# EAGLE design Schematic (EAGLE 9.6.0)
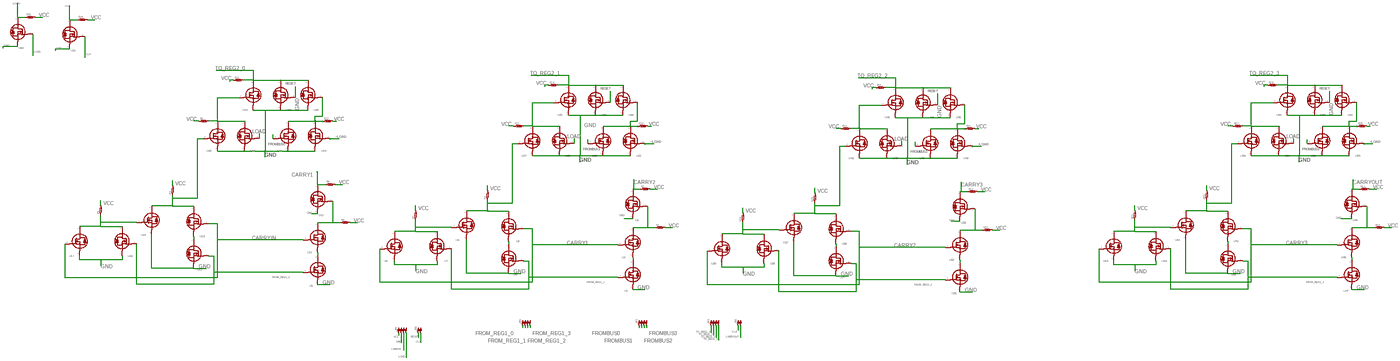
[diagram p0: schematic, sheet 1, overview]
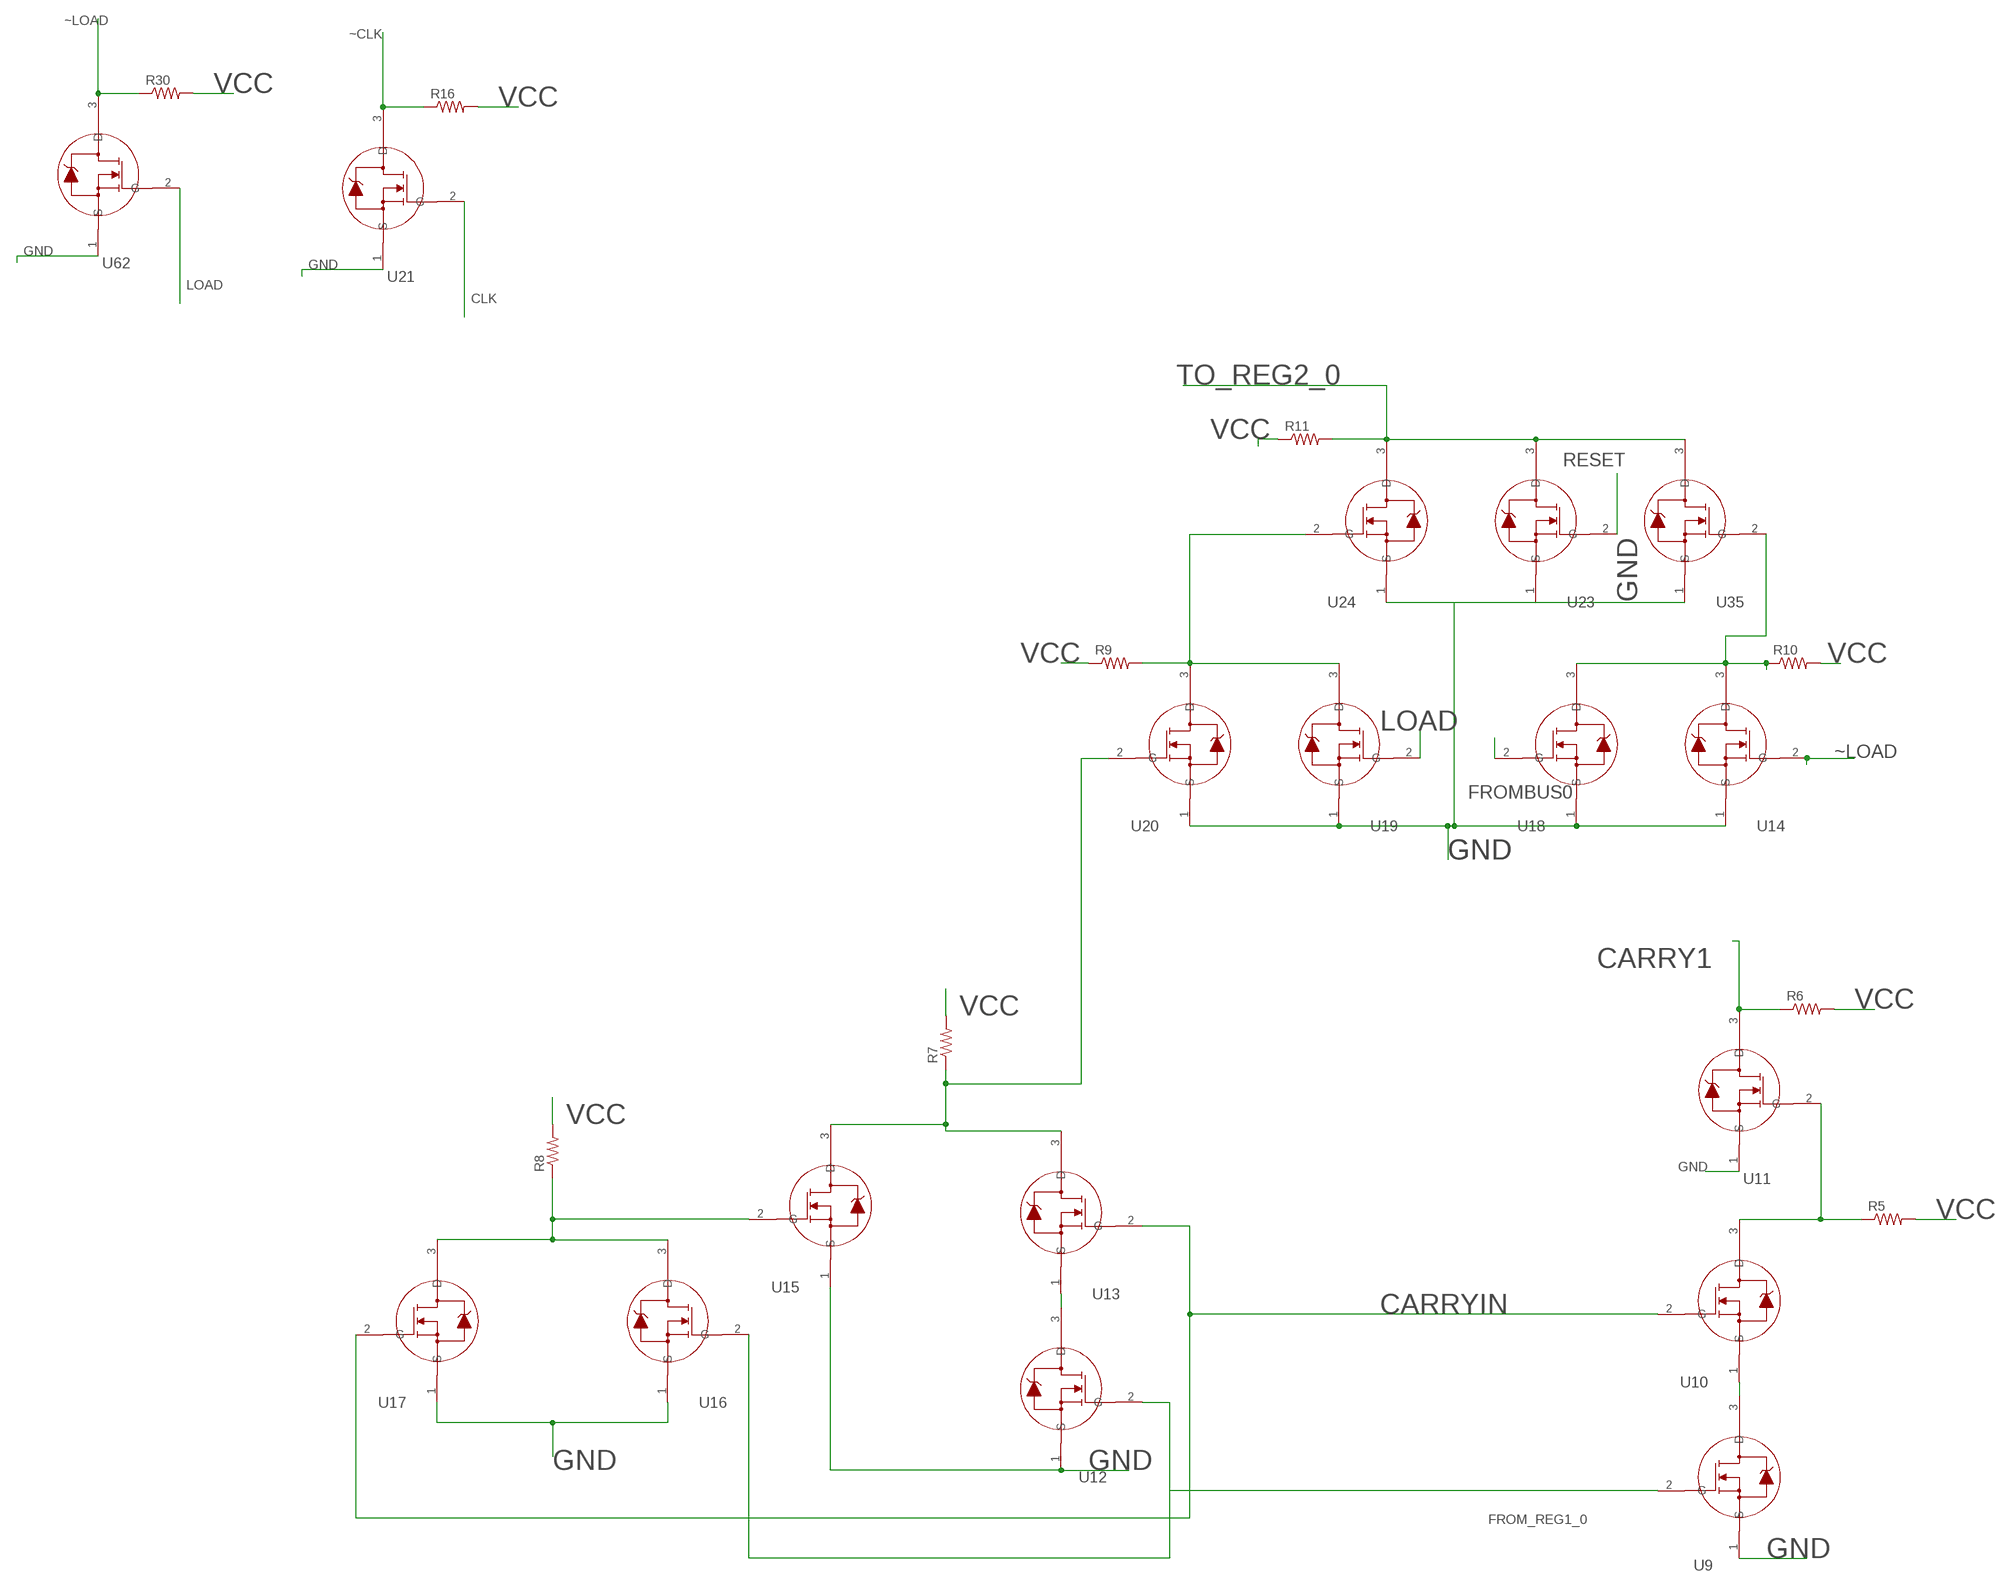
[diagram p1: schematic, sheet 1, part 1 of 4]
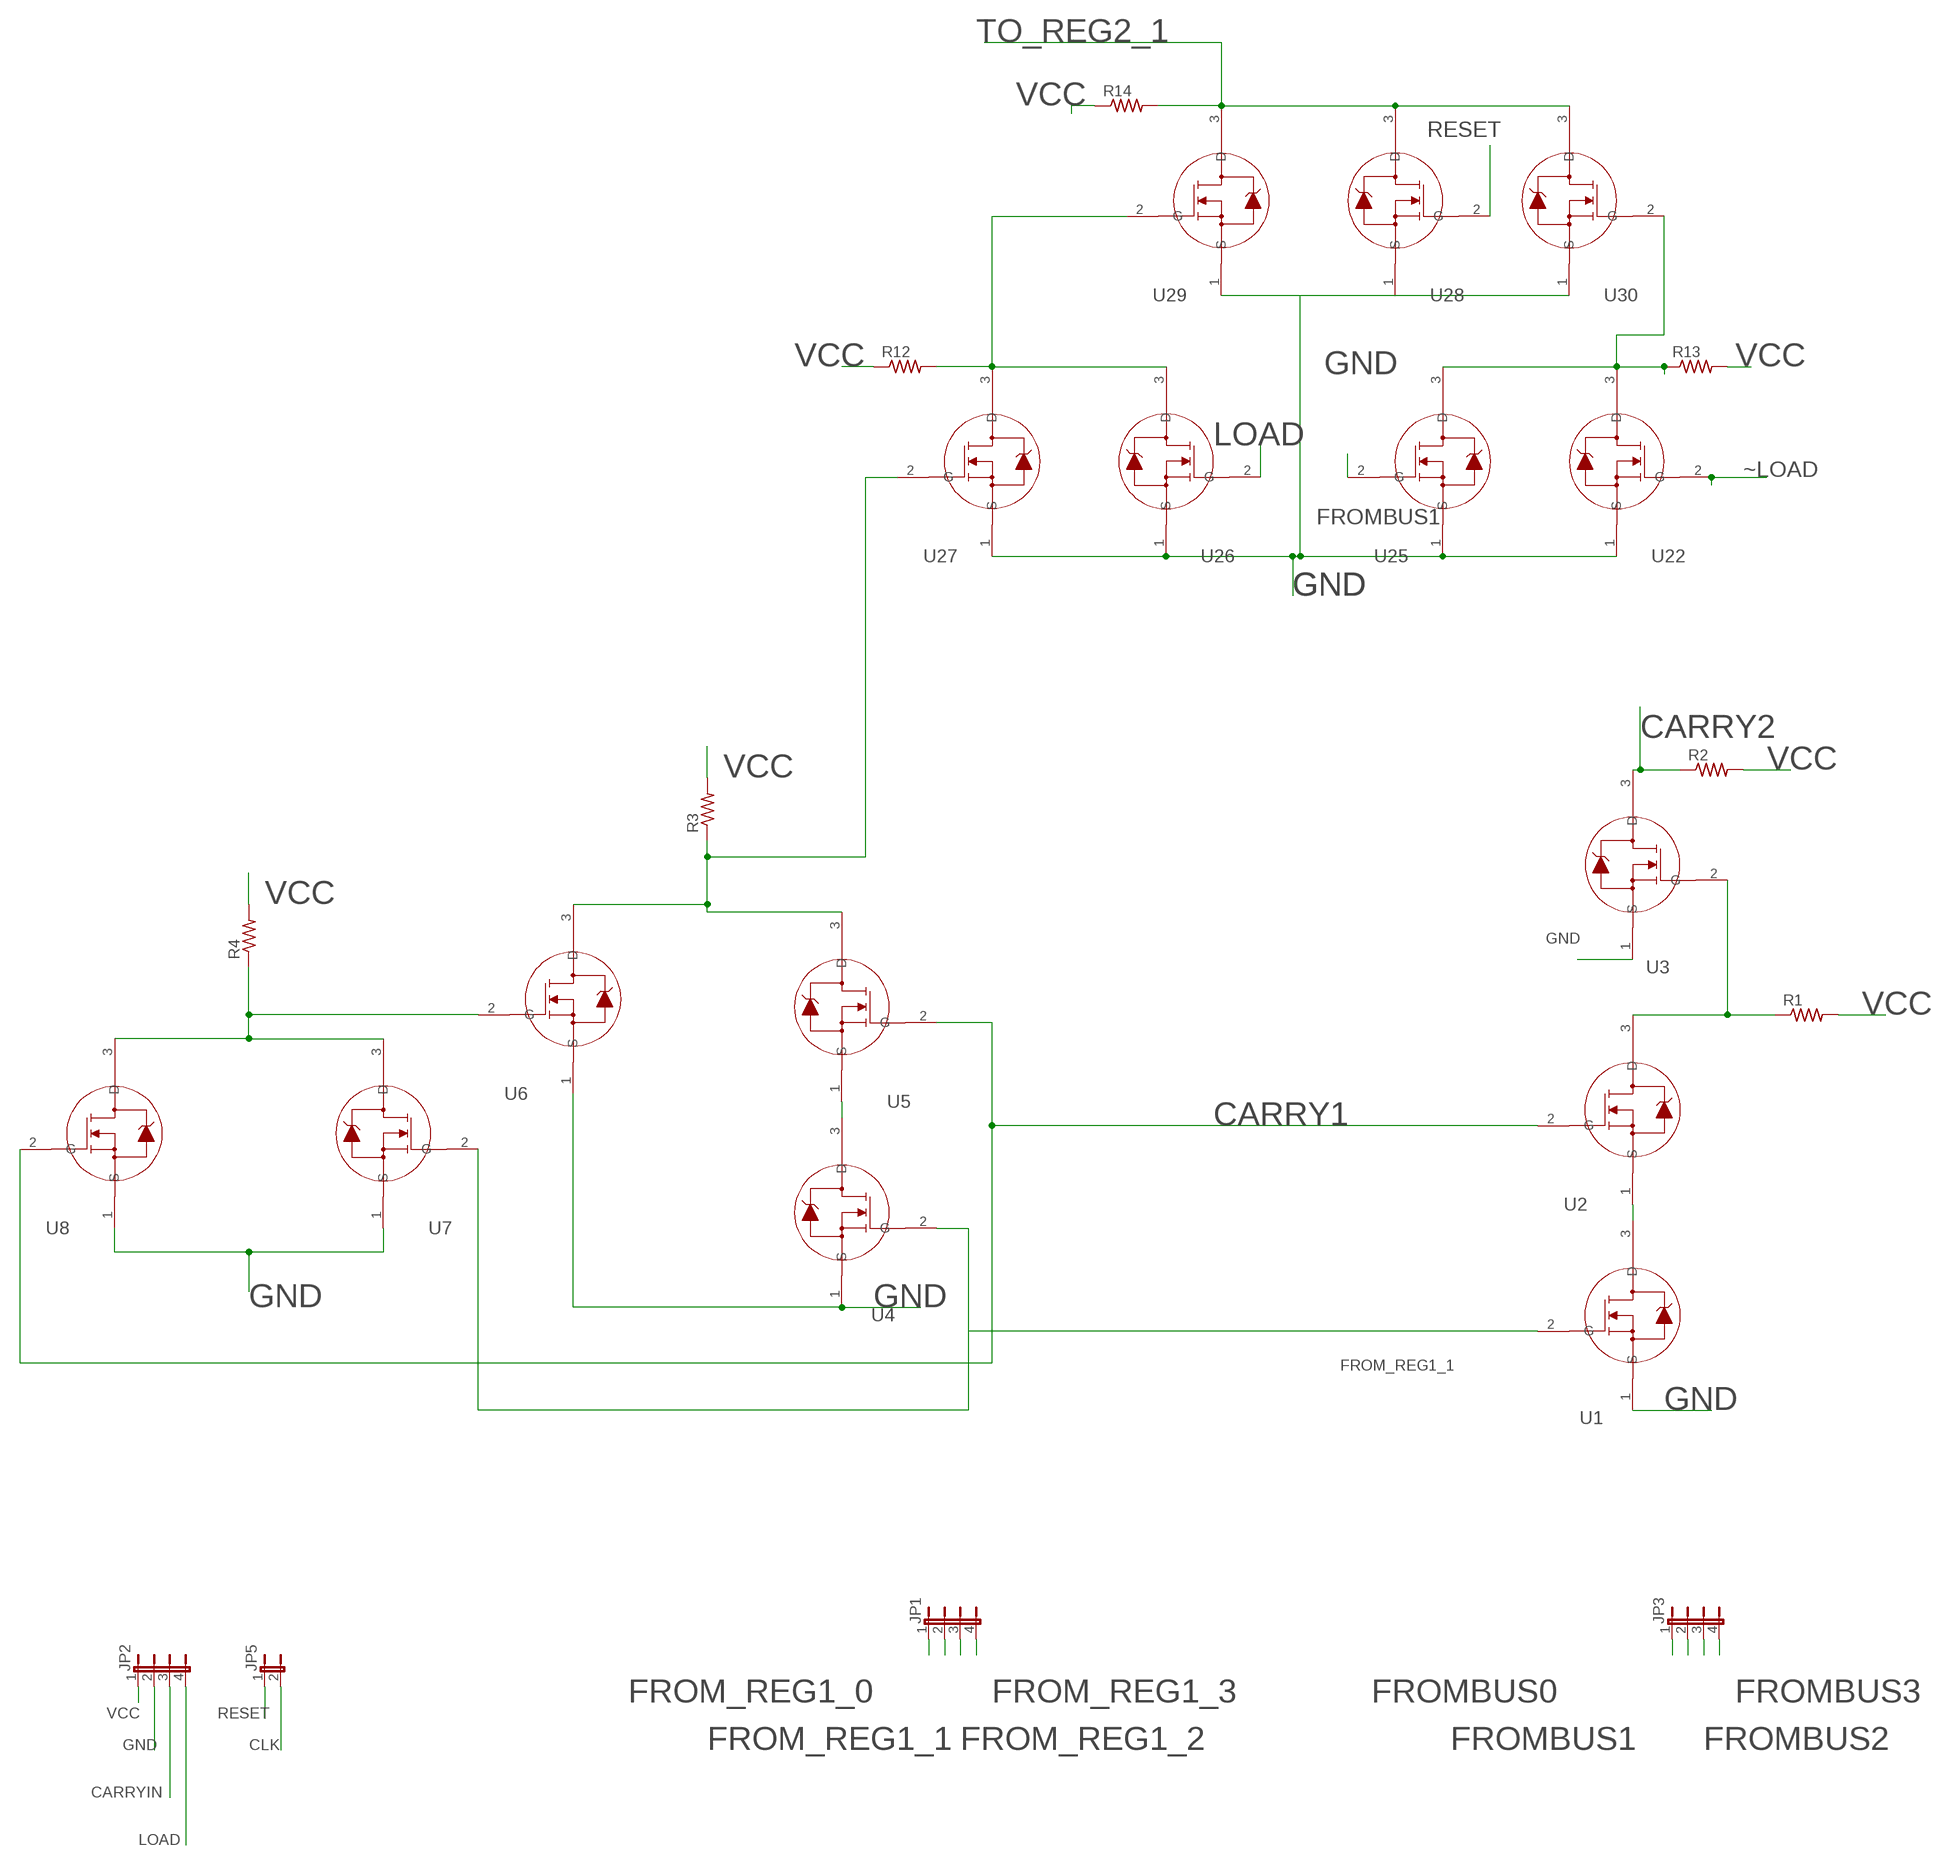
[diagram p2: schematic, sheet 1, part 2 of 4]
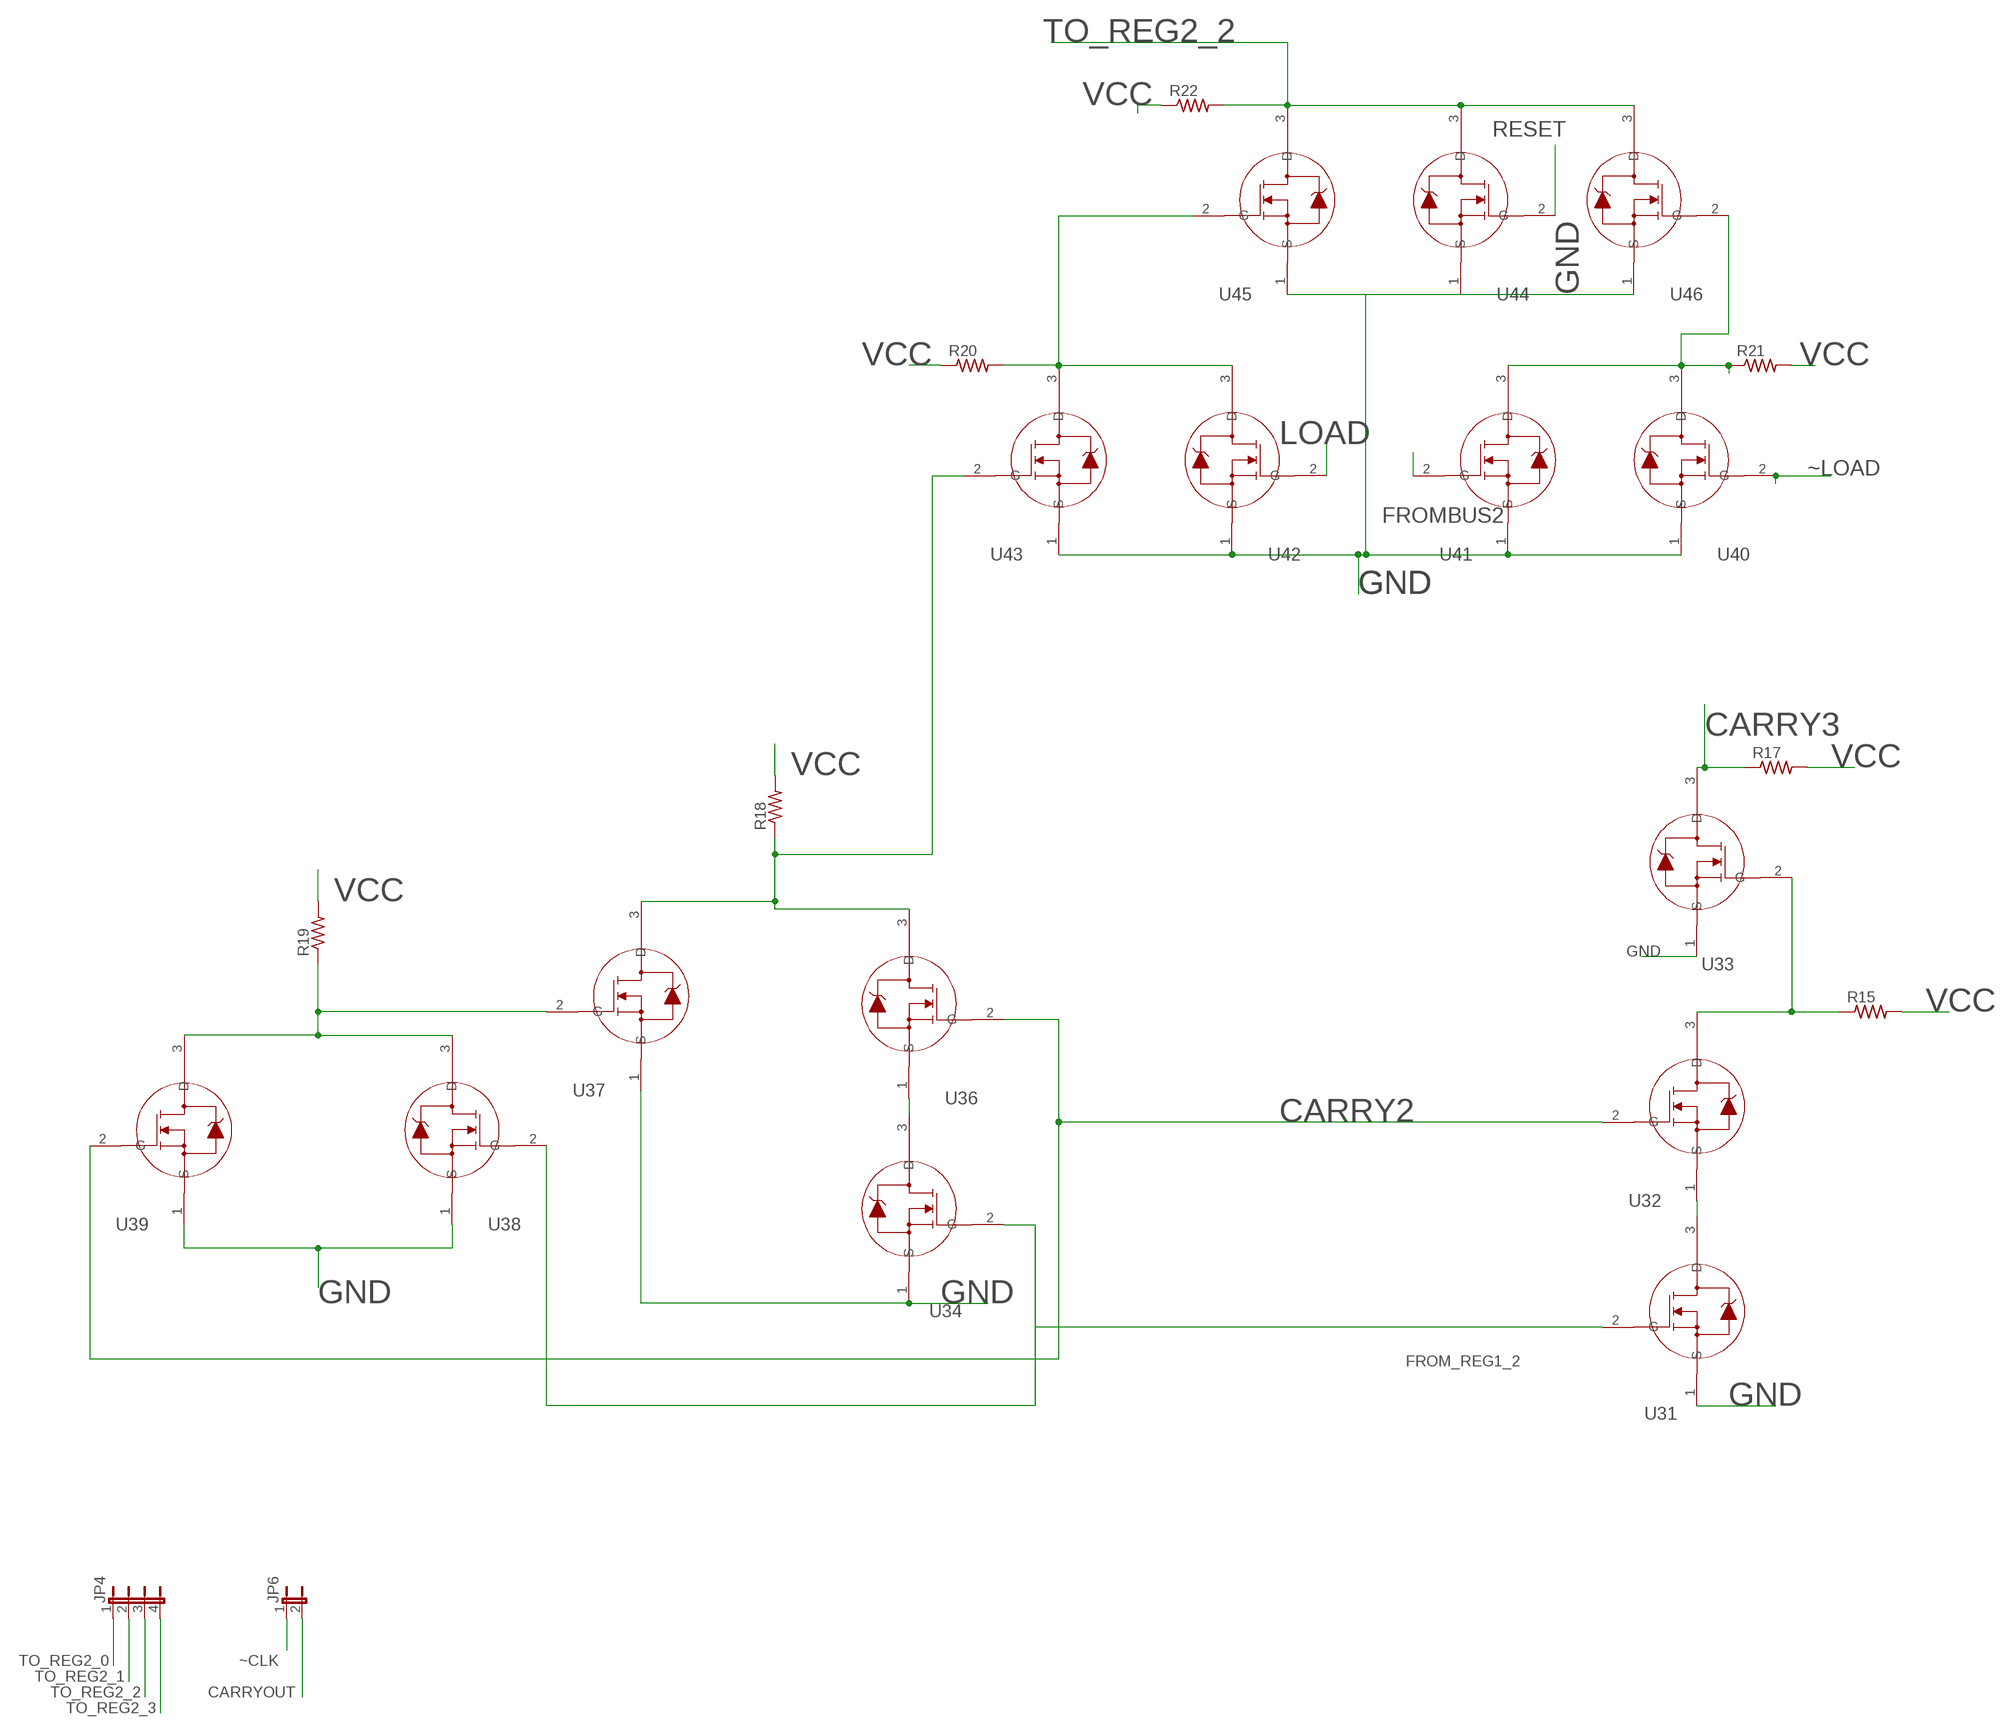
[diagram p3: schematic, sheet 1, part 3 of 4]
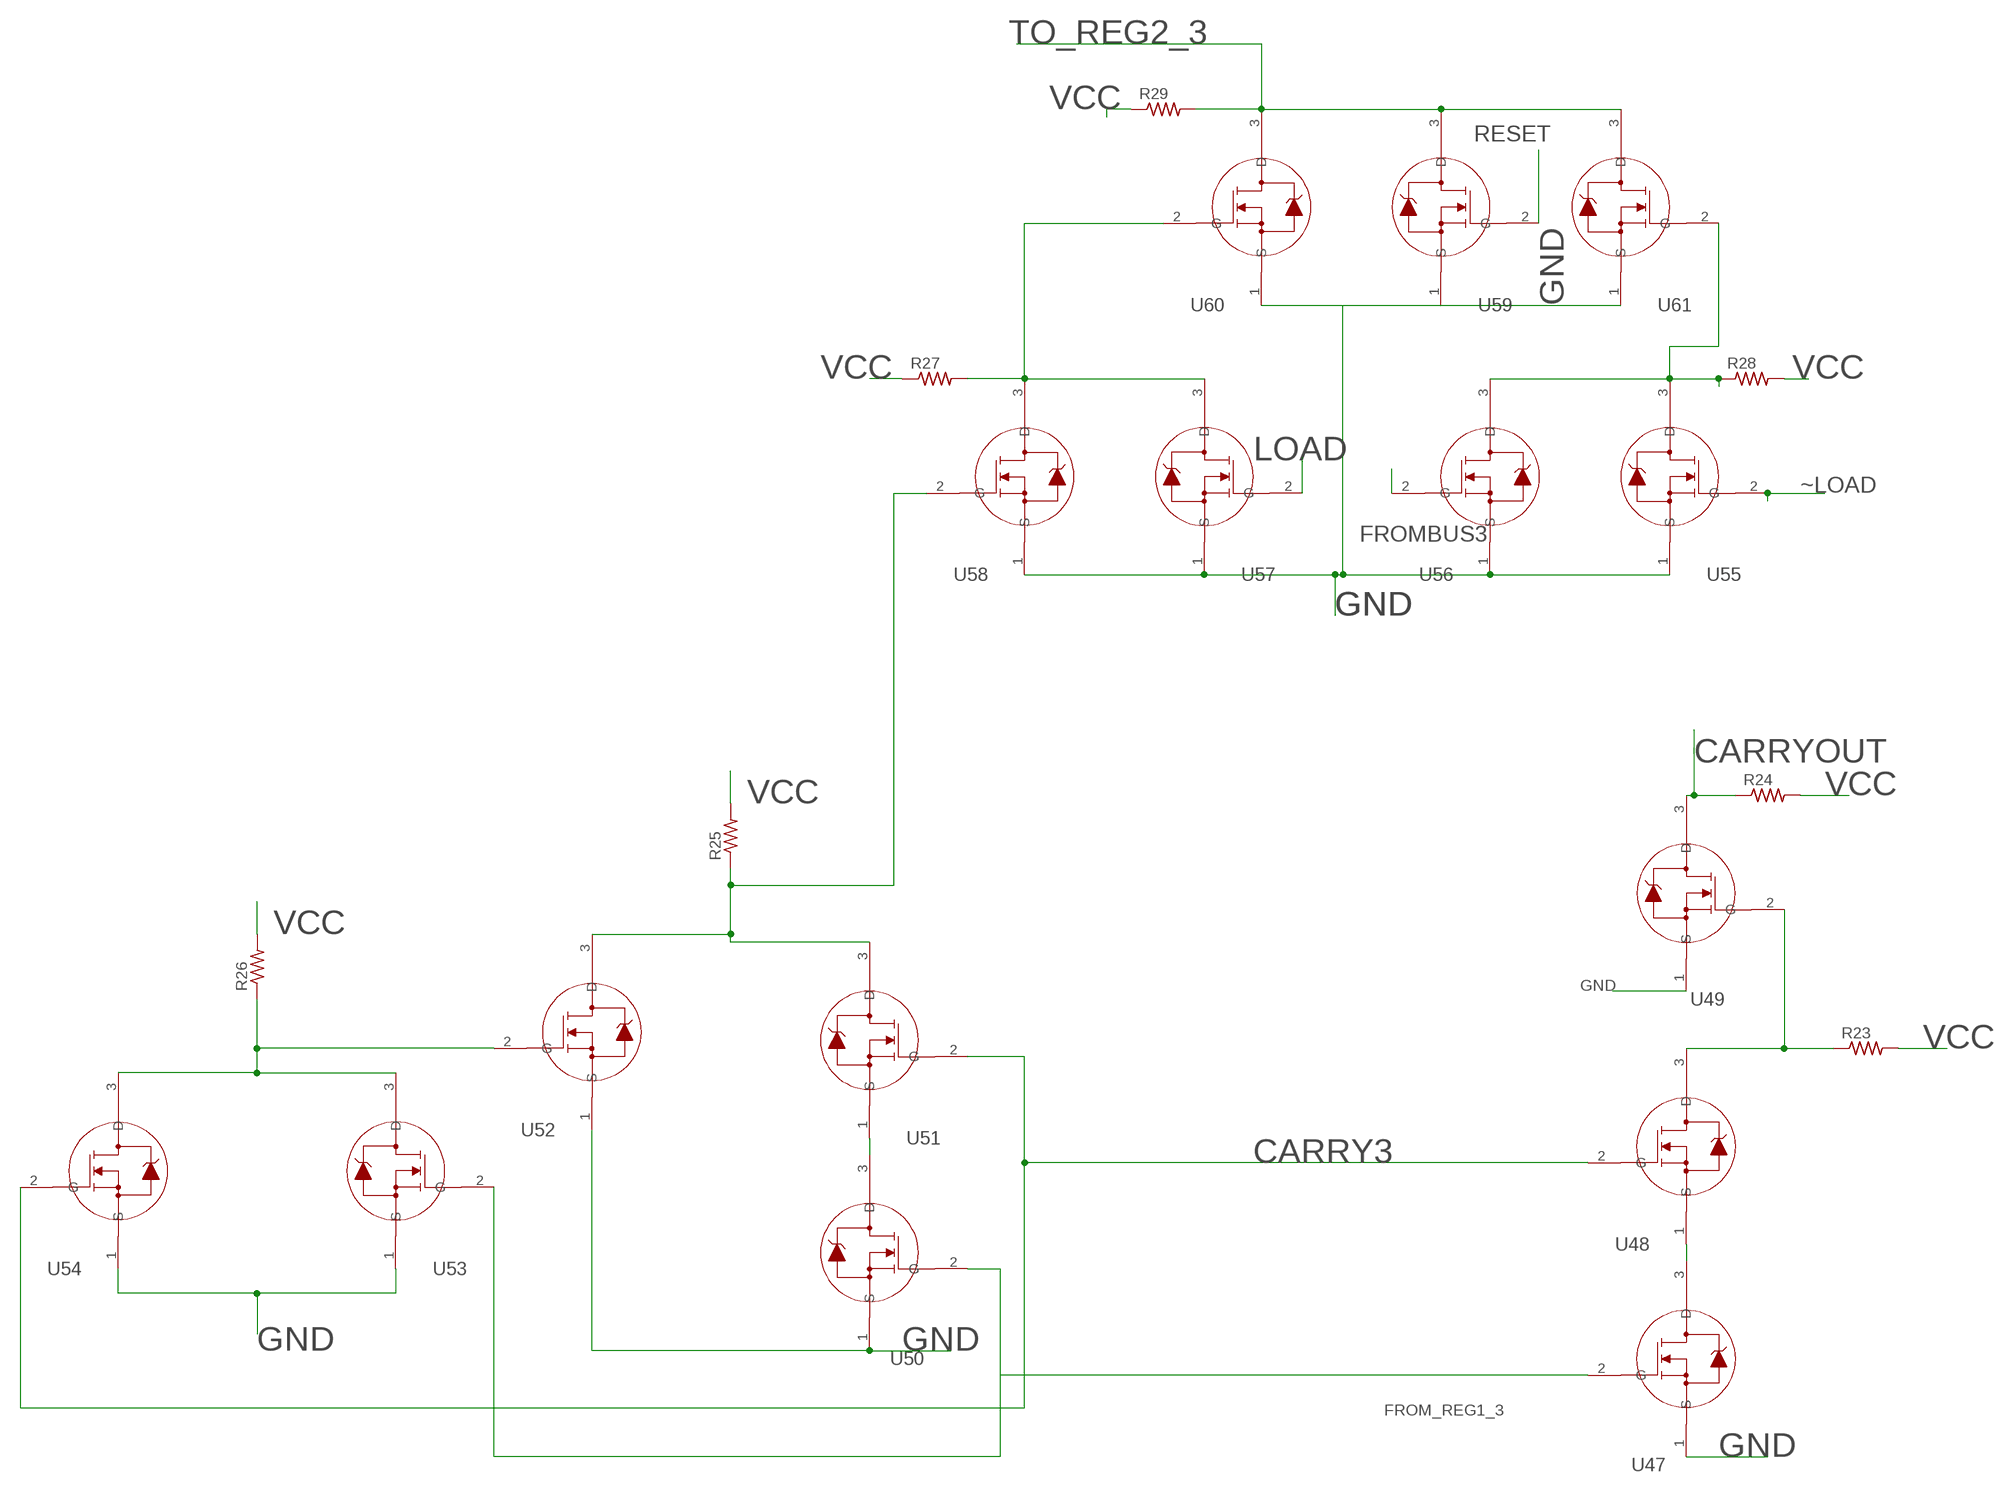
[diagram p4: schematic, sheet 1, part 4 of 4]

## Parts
JP1  JP4E  [JP4]
JP2  JP4E  [JP4]
JP3  JP4E  [JP4]
JP4  JP4E  [JP4]
JP5  JP1E  [JP1]
JP6  JP1E  [JP1]
R1  R-US_0204/7  [0204/7]
R2  R-US_0204/7  [0204/7]
R3  R-US_0204/7  [0204/7]
R4  R-US_0204/7  [0204/7]
R5  R-US_0204/7  [0204/7]
R6  R-US_0204/7  [0204/7]
R7  R-US_0204/7  [0204/7]
R8  R-US_0204/7  [0204/7]
R9  R-US_0204/7  [0204/7]
R10  R-US_0204/7  [0204/7]
R11  R-US_0204/7  [0204/7]
R12  R-US_0204/7  [0204/7]
R13  R-US_0204/7  [0204/7]
R14  R-US_0204/7  [0204/7]
R15  R-US_0204/7  [0204/7]
R16  R-US_0204/7  [0204/7]
R17  R-US_0204/7  [0204/7]
R18  R-US_0204/7  [0204/7]
R19  R-US_0204/7  [0204/7]
R20  R-US_0204/7  [0204/7]
R21  R-US_0204/7  [0204/7]
R22  R-US_0204/7  [0204/7]
R23  R-US_0204/7  [0204/7]
R24  R-US_0204/7  [0204/7]
R25  R-US_0204/7  [0204/7]
R26  R-US_0204/7  [0204/7]
R27  R-US_0204/7  [0204/7]
R28  R-US_0204/7  [0204/7]
R29  R-US_0204/7  [0204/7]
R30  R-US_0204/7  [0204/7]
U1  2N7000RLRAG  [TO-92_ONS]
U2  2N7000RLRAG  [TO-92_ONS]
U3  2N7000RLRAG  [TO-92_ONS]
U4  2N7000RLRAG  [TO-92_ONS]
U5  2N7000RLRAG  [TO-92_ONS]
U6  2N7000RLRAG  [TO-92_ONS]
U7  2N7000RLRAG  [TO-92_ONS]
U8  2N7000RLRAG  [TO-92_ONS]
U9  2N7000RLRAG  [TO-92_ONS]
U10  2N7000RLRAG  [TO-92_ONS]
U11  2N7000RLRAG  [TO-92_ONS]
U12  2N7000RLRAG  [TO-92_ONS]
U13  2N7000RLRAG  [TO-92_ONS]
U14  2N7000RLRAG  [TO-92_ONS]
U15  2N7000RLRAG  [TO-92_ONS]
U16  2N7000RLRAG  [TO-92_ONS]
U17  2N7000RLRAG  [TO-92_ONS]
U18  2N7000RLRAG  [TO-92_ONS]
U19  2N7000RLRAG  [TO-92_ONS]
U20  2N7000RLRAG  [TO-92_ONS]
U21  2N7000RLRAG  [TO-92_ONS]
U22  2N7000RLRAG  [TO-92_ONS]
U23  2N7000RLRAG  [TO-92_ONS]
U24  2N7000RLRAG  [TO-92_ONS]
U25  2N7000RLRAG  [TO-92_ONS]
U26  2N7000RLRAG  [TO-92_ONS]
U27  2N7000RLRAG  [TO-92_ONS]
U28  2N7000RLRAG  [TO-92_ONS]
U29  2N7000RLRAG  [TO-92_ONS]
U30  2N7000RLRAG  [TO-92_ONS]
U31  2N7000RLRAG  [TO-92_ONS]
U32  2N7000RLRAG  [TO-92_ONS]
U33  2N7000RLRAG  [TO-92_ONS]
U34  2N7000RLRAG  [TO-92_ONS]
U35  2N7000RLRAG  [TO-92_ONS]
U36  2N7000RLRAG  [TO-92_ONS]
U37  2N7000RLRAG  [TO-92_ONS]
U38  2N7000RLRAG  [TO-92_ONS]
U39  2N7000RLRAG  [TO-92_ONS]
U40  2N7000RLRAG  [TO-92_ONS]
U41  2N7000RLRAG  [TO-92_ONS]
U42  2N7000RLRAG  [TO-92_ONS]
U43  2N7000RLRAG  [TO-92_ONS]
U44  2N7000RLRAG  [TO-92_ONS]
U45  2N7000RLRAG  [TO-92_ONS]
U46  2N7000RLRAG  [TO-92_ONS]
U47  2N7000RLRAG  [TO-92_ONS]
U48  2N7000RLRAG  [TO-92_ONS]
U49  2N7000RLRAG  [TO-92_ONS]
U50  2N7000RLRAG  [TO-92_ONS]
U51  2N7000RLRAG  [TO-92_ONS]
U52  2N7000RLRAG  [TO-92_ONS]
U53  2N7000RLRAG  [TO-92_ONS]
U54  2N7000RLRAG  [TO-92_ONS]
U55  2N7000RLRAG  [TO-92_ONS]
U56  2N7000RLRAG  [TO-92_ONS]
U57  2N7000RLRAG  [TO-92_ONS]
U58  2N7000RLRAG  [TO-92_ONS]
U59  2N7000RLRAG  [TO-92_ONS]
U60  2N7000RLRAG  [TO-92_ONS]
U61  2N7000RLRAG  [TO-92_ONS]
U62  2N7000RLRAG  [TO-92_ONS]

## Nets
CARRY1: R6.1 U2.2(G) U5.2(G) U8.2(G) U11.3(D)
CARRY2: R2.1 U3.3(D) U32.2(G) U36.2(G) U39.2(G)
CARRY3: R17.1 U33.3(D) U48.2(G) U51.2(G) U54.2(G)
CARRYIN: JP2.3 U10.2(G) U13.2(G) U17.2(G)
CARRYOUT: JP6.2 R24.1 U49.3(D)
CLK: JP5.2 U21.2(G)
FROM_REG1_0: JP1.1 U9.2(G) U12.2(G) U16.2(G)
FROM_REG1_1: JP1.2 U1.2(G) U4.2(G) U7.2(G)
FROM_REG1_2: JP1.3 U31.2(G) U34.2(G) U38.2(G)
FROM_REG1_3: JP1.4 U47.2(G) U50.2(G) U53.2(G)
FROMBUS0: JP3.1 U18.2(G)
FROMBUS1: JP3.2 U25.2(G)
FROMBUS2: JP3.3 U41.2(G)
FROMBUS3: JP3.4 U56.2(G)
GND: JP2.2 U1.1(S) U3.1(S) U4.1(S) U6.1(S) U7.1(S) U8.1(S) U9.1(S) U11.1(S) U12.1(S) U14.1(S) U15.1(S) U16.1(S) U17.1(S) U18.1(S) U19.1(S) U20.1(S) U21.1(S) U22.1(S) U23.1(S) U24.1(S) U25.1(S) U26.1(S) U27.1(S) U28.1(S) U29.1(S) U30.1(S) U31.1(S) U33.1(S) U34.1(S) U35.1(S) U37.1(S) U38.1(S) U39.1(S) U40.1(S) U41.1(S) U42.1(S) U43.1(S) U44.1(S) U45.1(S) U46.1(S) U47.1(S) U49.1(S) U50.1(S) U52.1(S) U53.1(S) U54.1(S) U55.1(S) U56.1(S) U57.1(S) U58.1(S) U59.1(S) U60.1(S) U61.1(S) U62.1(S)
LOAD: JP2.4 U19.2(G) U26.2(G) U42.2(G) U57.2(G) U62.2(G)
N$1: U1.3(D) U2.1(S)
N$2: R1.1 U2.3(D) U3.2(G)
N$3: U31.3(D) U32.1(S)
N$4: U4.3(D) U5.1(S)
N$5: R3.1 U5.3(D) U6.3(D) U27.2(G)
N$6: R4.1 U6.2(G) U7.3(D) U8.3(D)
N$7: R12.2 U26.3(D) U27.3(D) U29.2(G)
N$8: R13.1 U22.3(D) U25.3(D) U30.2(G)
N$9: R9.2 U19.3(D) U20.3(D) U24.2(G)
N$10: U9.3(D) U10.1(S)
N$11: R15.1 U32.3(D) U33.2(G)
N$12: R5.1 U10.3(D) U11.2(G)
N$13: U12.3(D) U13.1(S)
N$15: R7.1 U13.3(D) U15.3(D) U20.2(G)
N$16: R8.1 U15.2(G) U16.3(D) U17.3(D)
N$17: R10.1 U14.3(D) U18.3(D) U35.2(G)
N$18: U47.3(D) U48.1(S)
N$19: R23.1 U48.3(D) U49.2(G)
N$20: U34.3(D) U36.1(S)
N$21: R18.1 U36.3(D) U37.3(D) U43.2(G)
N$22: R19.1 U37.2(G) U38.3(D) U39.3(D)
N$23: R20.2 U42.3(D) U43.3(D) U45.2(G)
N$24: R21.1 U40.3(D) U41.3(D) U46.2(G)
N$25: U50.3(D) U51.1(S)
N$26: R25.1 U51.3(D) U52.3(D) U58.2(G)
N$27: R26.1 U52.2(G) U53.3(D) U54.3(D)
N$28: R27.2 U57.3(D) U58.3(D) U60.2(G)
N$29: R28.1 U55.3(D) U56.3(D) U61.2(G)
RESET: JP5.1 U23.2(G) U28.2(G) U44.2(G) U59.2(G)
TO_REG2_0: JP4.1 R11.2 U23.3(D) U24.3(D) U35.3(D)
TO_REG2_1: JP4.2 R14.2 U28.3(D) U29.3(D) U30.3(D)
TO_REG2_2: JP4.3 R22.2 U44.3(D) U45.3(D) U46.3(D)
TO_REG2_3: JP4.4 R29.2 U59.3(D) U60.3(D) U61.3(D)
VCC: JP2.1 R1.2 R2.2 R3.2 R4.2 R5.2 R6.2 R7.2 R8.2 R9.1 R10.2 R11.1 R12.1 R13.2 R14.1 R15.2 R16.2 R17.2 R18.2 R19.2 R20.1 R21.2 R22.1 R23.2 R24.2 R25.2 R26.2 R27.1 R28.2 R29.1 R30.2
~CLK: JP6.1 R16.1 U21.3(D)
~LOAD: R30.1 U14.2(G) U22.2(G) U40.2(G) U55.2(G) U62.3(D)

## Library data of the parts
JP1-JP4 = jumper:JP4E: JUMPER
JP5 JP6 = jumper:JP1E: JUMPER
R1-R30 = rcl:R-US_: RESISTOR, American symbol; SPICEPREFIX: R
U1-U62 = Transistor(MOSFET):2N7000RLRAG; COPYRIGHT: Copyright (C) 2022 Ultra Librarian. All rights reserved.; MANUFACTURER_PART_NUMBER: 2N7000RLRAG; MFR_NAME: onsemi

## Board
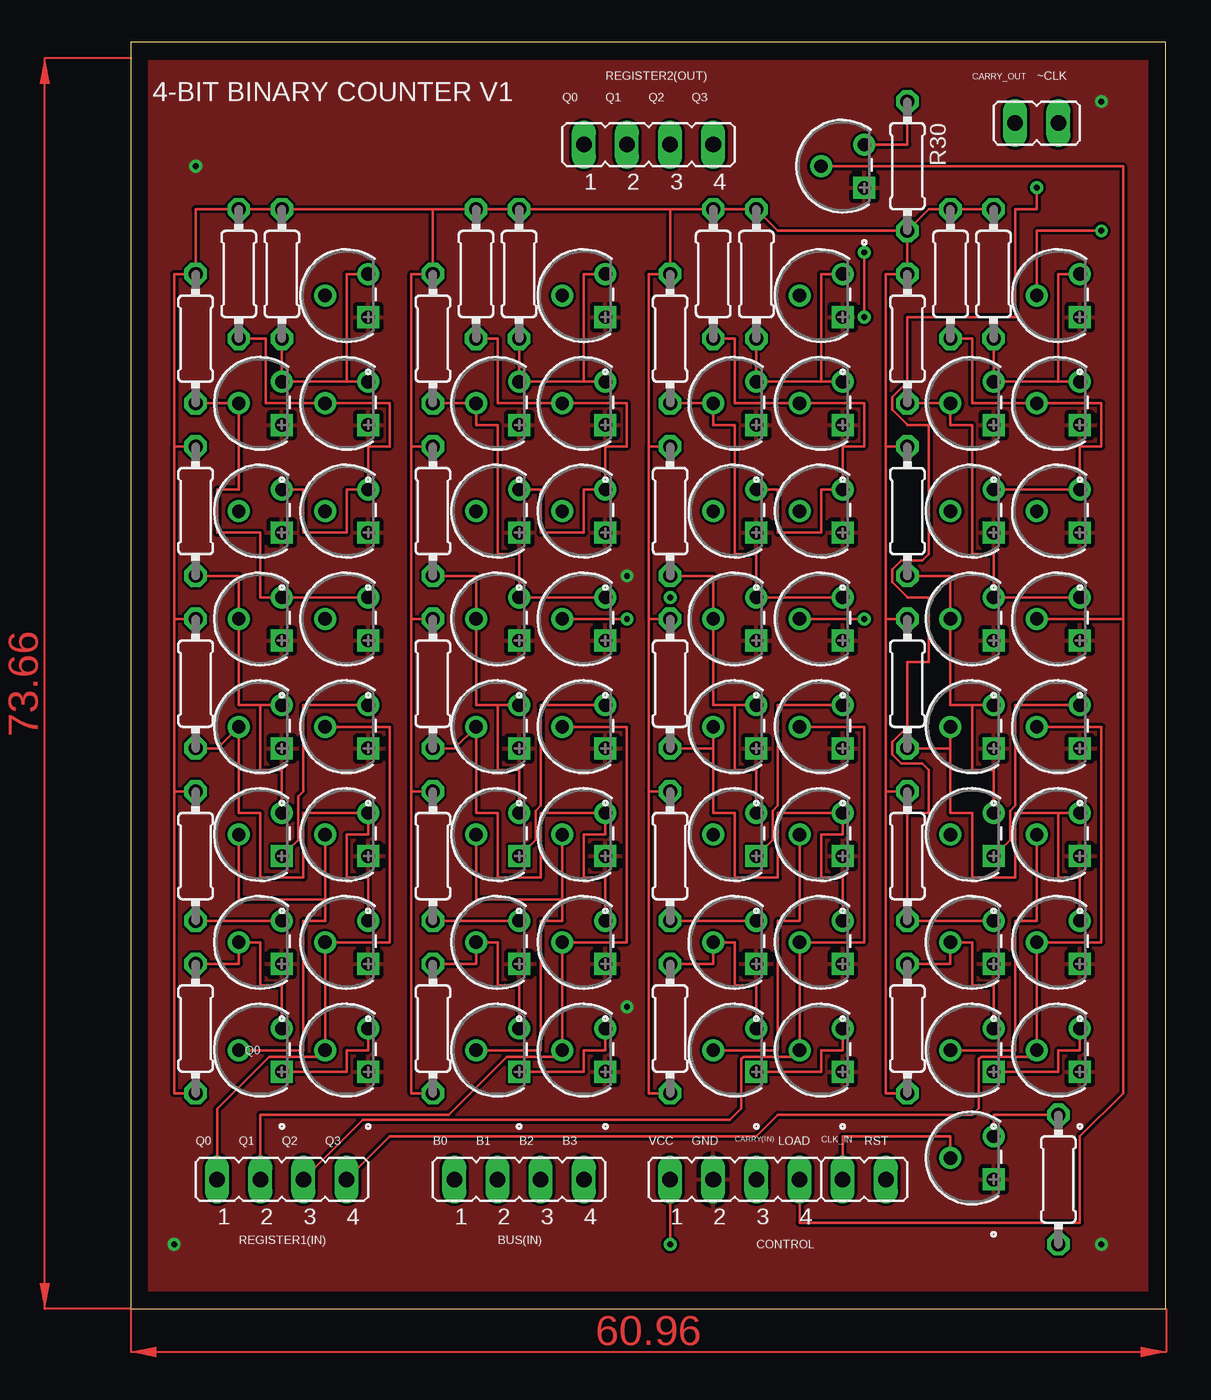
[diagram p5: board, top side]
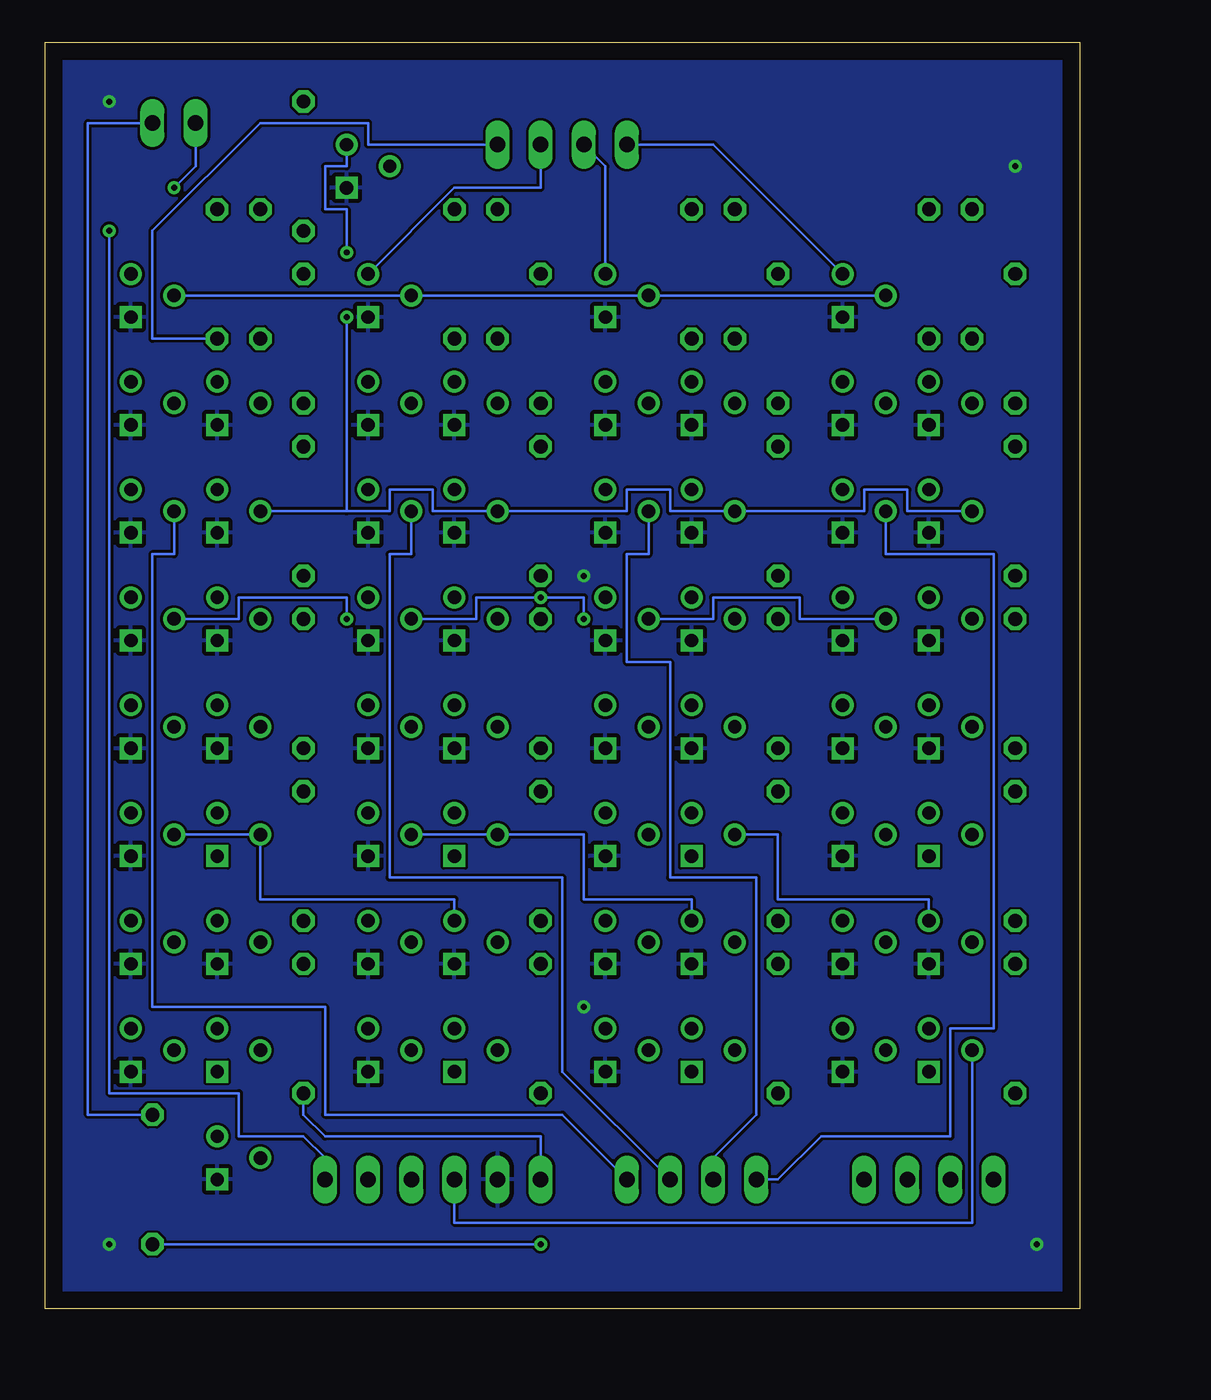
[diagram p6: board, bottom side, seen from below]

Size 60.94 x 74.6 mm. Coordinates in mm from the lower left corner, seen from the top.
Outline: 0,0 60.94,0 60.94,74.6 0,74.6 0,0
Copper layers (1*16): Top 0.035mm / dielectric 1.5mm / Bottom 0.035mm
Design rules "default": minimum track width 6mil, minimum drill 0.35mm, track to track 6mil, track to pad 6mil, pad to pad 6mil, via to via 6mil, smd to smd 6mil, copper to edge 40mil, drill to drill 6mil, minimum pad ring 10mil, minimum via ring 8mil, stop-mask expansion 4mil, vias tented up to drill 0mil, thermal gap 10mil

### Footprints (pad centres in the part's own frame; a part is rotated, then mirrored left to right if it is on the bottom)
JP4 = drill 0.914 long: 1 -3.81,0; 2 -1.27,0; 3 1.27,0; 4 3.81,0
JP1 = drill 0.914 long: 1 0,-1.27; 2 0,1.27
0204/7 = drill 0.813 octagon: 1 -3.81,0; 2 3.81,0
TO-92_ONS = drill 0.787 pad 1.295 square: 1 0,0 | drill 0.787 pad 1.295: 2 1.27,2.54; 3 2.54,0

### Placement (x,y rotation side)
JP1  8.89,7.62 0 top
JP2  35.56,7.62 0 top
JP3  22.86,7.62 0 top
JP4  30.48,68.58 0 top
JP5  43.18,7.62 90 top
JP6  53.34,69.85 90 top
R1  17.78,16.51 270 top
R2  17.78,26.67 90 top
R3  17.78,46.99 90 top
R4  17.78,36.83 90 top
R5  3.81,16.51 270 top
R6  3.81,26.67 90 top
R7  3.81,46.99 90 top
R8  3.81,36.83 90 top
R9  3.81,57.15 270 top
R10  6.35,60.96 90 top
R11  8.89,60.96 270 top
R12  17.78,57.15 270 top
R13  20.32,60.96 90 top
R14  22.86,60.96 270 top
R15  31.75,16.51 270 top
R16  54.61,7.62 270 top
R17  31.75,26.67 90 top
R18  31.75,46.99 90 top
R19  31.75,36.83 90 top
R20  31.75,57.15 270 top
R21  34.29,60.96 90 top
R22  36.83,60.96 270 top
R23  45.72,16.51 270 top
R24  45.72,26.67 90 top
R25  45.72,46.99 90 top
R26  45.72,36.83 90 top
R27  45.72,57.15 270 top
R28  48.26,60.96 90 top
R29  50.8,60.96 270 top
R30  45.72,67.31 270 top
U1  27.94,13.97 90 top
U2  22.86,13.97 90 top
U3  22.86,20.32 90 top
U4  27.94,33.02 90 top
U5  22.86,26.67 90 top
U6  22.86,33.02 90 top
U7  27.94,20.32 90 top
U8  27.94,26.67 90 top
U9  13.97,13.97 90 top
U10  8.89,13.97 90 top
U11  8.89,20.32 90 top
U12  13.97,33.02 90 top
U13  8.89,26.67 90 top
U14  8.89,45.72 90 top
U15  8.89,33.02 90 top
U16  13.97,20.32 90 top
U17  13.97,26.67 90 top
U18  13.97,45.72 90 top
U19  13.97,39.37 90 top
U20  8.89,39.37 90 top
U21  50.8,7.62 90 top
U22  22.86,45.72 90 top
U23  13.97,58.42 90 top
U24  8.89,52.07 90 top
U25  27.94,45.72 90 top
U26  27.94,39.37 90 top
U27  22.86,39.37 90 top
U28  27.94,58.42 90 top
U29  22.86,52.07 90 top
U30  27.94,52.07 90 top
U31  41.91,13.97 90 top
U32  36.83,13.97 90 top
U33  36.83,20.32 90 top
U34  41.91,33.02 90 top
U35  13.97,52.07 90 top
U36  36.83,26.67 90 top
U37  36.83,33.02 90 top
U38  41.91,20.32 90 top
U39  41.91,26.67 90 top
U40  36.83,45.72 90 top
U41  41.91,45.72 90 top
U42  41.91,39.37 90 top
U43  36.83,39.37 90 top
U44  41.91,58.42 90 top
U45  36.83,52.07 90 top
U46  41.91,52.07 90 top
U47  55.88,13.97 90 top
U48  50.8,13.97 90 top
U49  50.8,20.32 90 top
U50  55.88,33.02 90 top
U51  50.8,26.67 90 top
U52  50.8,33.02 90 top
U53  55.88,20.32 90 top
U54  55.88,26.67 90 top
U55  50.8,45.72 90 top
U56  55.88,45.72 90 top
U57  55.88,39.37 90 top
U58  50.8,39.37 90 top
U59  55.88,58.42 90 top
U60  50.8,52.07 90 top
U61  55.88,52.07 90 top
U62  43.18,66.04 90 top

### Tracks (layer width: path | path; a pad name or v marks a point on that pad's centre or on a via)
CARRY1
  Top 0.152: U2.2 24.13,15.24 24.13,22.86 25.4,22.86 25.4,24.13 | 25.4,24.13 U8.2 | 25.4,24.13 20.32,24.13 U5.2 | R6.1 U11.3
  Bottom 0.152: U11.3 8.89,24.13 17.78,24.13 17.78,27.94 U5.2
CARRY2
  Top 0.152: R2.1 U3.3 | U39.2 39.37,22.86 38.1,22.86 38.1,15.24 U32.2
  Bottom 0.152: U39.2 U36.2 29.21,27.94 29.21,24.13 22.86,24.13 U3.3
CARRY3
  Top 0.152: R17.1 U33.3 | U48.2 52.07,15.24 52.07,22.86 53.34,22.86 U54.2
  Bottom 0.152: U33.3 36.83,24.13 48.26,24.13 U51.2 U54.2
CARRYIN
  Top 0.152: U10.2 10.16,15.24 10.16,22.86 11.43,22.86 11.43,24.13 | U17.2 11.43,24.13 | U13.2 6.35,24.13 11.43,24.13
  Bottom 0.152: JP2.3 36.83,5.08 6.35,5.08 U10.2
CARRYOUT  (via drill 0.35)
  Top 0.152: U49.3 R24.1 45.72,29.21 46.99,29.21 46.99,31.75 46.61,32.13 45.35,32.13 44.83,32.65 44.83,33.39 45.72,34.28 45.72,38.1 46.99,38.1 46.99,41.91 45.72,41.91 45.72,41.92 44.83,42.81 44.83,43.55 45.35,44.07 46.61,44.07 46.99,44.45 46.99,52.07 45.72,52.07 45.72,52.08 44.83,52.97 44.83,53.71 45.72,54.6 45.72,58.42 52.07,58.42 52.07,64.77 53.34,64.77 v53.34,66.04
  Bottom 0.152: JP6.2 52.07,67.31 v53.34,66.04
CLK
  Top 0.152: JP5.2 41.91,10.16 48.26,10.16 U21.2
FROM_REG1_0
  Top 0.152: U12.2 15.24,34.29 15.24,21.59 U16.2 U9.2 11.04,14.85 8.15,14.85 5.08,11.78 JP1.1
FROM_REG1_1
  Top 0.152: U4.2 29.21,34.29 29.21,21.59 U7.2 U1.2 25.01,14.85 22.12,14.85 18.7,11.43 7.62,11.43 JP1.2
FROM_REG1_2
  Top 0.152: U34.2 43.18,34.29 43.18,21.59 U38.2 U31.2 38.98,14.85 36.09,14.85 35.95,14.71 35.95,11.82 35.25,11.12 13.67,11.12 JP1.3
FROM_REG1_3
  Top 0.152: U50.2 57.15,34.29 57.15,21.59 U53.2 U47.2 52.95,14.85 50.06,14.85 49.92,14.71 49.92,11.82 49.53,11.43 38.1,11.43 36.83,10.16 15.24,10.16 JP1.4
FROMBUS0
  Bottom 0.152: JP3.1 17.78,7.62 15.24,10.16 7.62,10.16 7.62,16.51 5.08,16.51 5.08,44.45 11.43,44.45 U18.2
FROMBUS1
  Bottom 0.152: JP3.2 21.59,8.89 19.05,11.43 19.05,25.4 24.13,25.4 24.13,38.1 26.67,38.1 26.67,44.45 25.4,44.45 U25.2
FROMBUS2
  Bottom 0.152: U41.2 39.37,44.45 40.64,44.45 40.64,25.4 30.48,25.4 30.48,13.97 JP3.3
FROMBUS3
  Bottom 0.152: JP3.4 30.48,11.43 44.45,11.43 44.45,17.78 54.61,17.78 54.61,44.45 53.34,44.45 U56.2
GND  (via drill 0.35)
  other vias: 29.21,17.78 2.54,3.81 57.15,3.81 3.81,67.31 57.15,71.12 29.21,43.18
  pour Top: -1.27,73.66 60.96,73.66 60.96,-1.27 -1.27,-1.27
  pour Bottom: -1.27,73.66 60.96,73.66 60.96,-1.27 -1.27,-1.27
LOAD  (via drill 0.35)
  Top 0.152: U26.2 v29.21,40.64 | U42.2 v43.18,40.64 | U62.2 58.42,67.31 58.42,40.64 | 58.42,40.64 58.42,12.7 55.88,10.16 55.88,5.08 39.37,5.08 JP2.4 | U57.2 58.42,40.64
  Bottom 0.152: U42.2 35.56,40.64 35.56,41.91 v31.75,41.91 29.21,41.91 v29.21,40.64 | U19.2 16.51,40.64 16.51,41.91 21.59,41.91 21.59,40.64 U26.2 | v43.18,40.64 43.18,41.91 49.53,41.91 49.53,40.64 U57.2
N$1
  Top 0.152: U2.1 26.67,13.97 26.67,15.24 27.94,15.24 U1.3
N$2
  Top 0.152: U2.3 22.86,19.05 21.59,19.05 21.59,21.59 U3.2 20.32,20.32 R1.1
N$3
  Top 0.152: U32.1 40.64,13.97 40.64,15.24 41.91,15.24 U31.3
N$4
  Top 0.152: U4.3 24.13,35.56 24.13,29.64 23.82,29.34 23.82,27.64 U5.1
N$5
  Top 0.152: 21.59,35.56 20.32,35.56 U27.2 20.32,43.18 R3.1 | 21.59,35.56 U6.3 | 21.59,35.56 21.59,31.75 22.86,31.75 U5.3
N$6
  Top 0.152: U7.3 27.94,25.4 26.67,25.4 26.67,27.94 27.94,27.94 U8.3 24.13,29.21 24.13,25.4 21.59,25.4 21.59,29.21 20.32,29.21 U6.2 19.05,33.02 R4.1
N$7
  Top 0.152: U26.3 U27.3 22.86,44.45 21.59,44.45 21.59,52.07 20.32,52.07 U29.2 R12.2
N$8
  Top 0.152: U22.3 24.13,48.26 24.13,45.72 26.67,45.72 26.67,48.26 U25.3 27.94,50.8 29.21,50.8 29.21,53.34 U30.2 21.59,53.34 21.59,57.15 R13.1
N$9
  Top 0.152: U19.3 U20.3 7.62,41.91 7.62,45.72 5.08,45.72 5.08,48.26 6.35,48.26 U24.2 R9.2
N$10
  Top 0.152: U10.1 12.7,13.97 12.7,15.24 13.97,15.24 U9.3
N$11
  Top 0.152: U32.3 36.83,19.05 35.56,19.05 35.56,21.59 U33.2 34.29,20.32 R15.1
N$12
  Top 0.152: U10.3 8.89,19.05 7.62,19.05 7.62,21.59 U11.2 6.35,20.32 R5.1
N$13
  Top 0.152: U13.1 9.86,27.64 9.86,30.18 10.16,30.48 10.16,35.56 U12.3
N$15
  Top 0.152: U13.3 8.89,31.75 7.62,31.75 7.62,35.56 | U15.3 7.62,35.56 | 7.62,35.56 6.35,35.56 U20.2 6.35,43.18 R7.1
N$16
  Top 0.152: U16.3 13.97,25.4 12.7,25.4 12.7,27.94 13.97,27.94 U17.3 10.16,29.21 10.16,25.4 7.62,25.4 7.62,29.21 6.35,29.21 U15.2 5.08,33.02 R8.1
N$17
  Top 0.152: U14.3 10.16,48.26 10.16,45.72 12.7,45.72 12.7,48.26 U18.3 13.97,50.8 15.24,50.8 15.24,53.34 U35.2 7.93,53.34 7.93,57.15 R10.1
N$18
  Top 0.152: U48.1 54.61,13.97 54.61,15.24 55.88,15.24 U47.3
N$19
  Top 0.152: U48.3 50.8,19.05 49.53,19.05 49.53,21.59 U49.2 48.26,20.32 R23.1
N$20
  Top 0.152: U34.3 38.1,35.56 38.1,29.64 37.8,29.34 37.8,27.64 U36.1
N$21
  Top 0.152: U37.3 35.56,35.56 | 35.56,35.56 34.29,35.56 U43.2 34.29,43.18 R18.1 | U36.3 36.83,31.75 35.56,31.75 35.56,35.56
N$22
  Top 0.152: U38.3 41.91,25.4 40.64,25.4 40.64,27.94 41.91,27.94 U39.3 38.1,29.21 38.1,25.4 35.56,25.4 35.56,29.21 34.29,29.21 34.29,33.02 | U37.2 34.29,33.02 | R19.1 34.29,33.02
N$23
  Top 0.152: U42.3 U43.3 36.83,44.45 35.56,44.45 35.56,52.07 34.29,52.07 U45.2 R20.2
N$24
  Top 0.152: U40.3 38.1,48.26 38.1,45.72 40.64,45.72 40.64,48.26 U41.3 41.91,50.8 43.18,50.8 43.18,53.34 U46.2 35.56,53.34 35.56,57.15 R21.1
N$25
  Top 0.152: U50.3 52.07,35.56 52.07,29.64 51.77,29.34 51.77,27.64 U51.1
N$26
  Top 0.152: 49.53,35.56 48.26,35.56 U58.2 48.26,43.18 R25.1 | 49.53,35.56 U52.3 | U51.3 50.8,31.75 49.53,31.75 49.53,35.56
N$27
  Top 0.152: U52.2 48.26,33.02 | 48.26,33.02 48.26,29.21 49.53,29.21 49.53,25.4 52.07,25.4 52.07,29.21 54.61,29.21 | 54.61,29.21 U54.3 | U53.3 55.88,25.4 54.61,25.4 54.61,29.21 | R26.1 48.26,33.02
N$28
  Top 0.152: U57.3 U58.3 50.8,44.45 49.53,44.45 49.53,52.07 48.26,52.07 U60.2 R27.2
N$29
  Top 0.152: U55.3 U56.3 55.88,50.8 57.15,50.8 57.15,53.34 U61.2 49.53,53.34 49.53,57.15 R28.1
RESET  (via drill 0.35)
  Top 0.152: U59.2 53.34,63.5 v57.15,63.5
  Bottom 0.152: U23.2 U28.2 U44.2 U59.2 | JP5.1 44.45,8.89 45.72,10.16 49.53,10.16 49.53,11.43 | v57.15,63.5 57.15,12.7 49.53,12.7 49.53,11.43 | 49.53,11.43
TO_REG2_0
  Top 0.152: 12.7,54.61 U24.3 R11.2 | 12.7,54.61 12.7,60.96 U23.3 | U35.3 12.7,54.61
  Bottom 0.152: U23.3 21.59,68.58 JP4.1
TO_REG2_1
  Top 0.152: 26.67,54.61 U29.3 R14.2 | 26.67,54.61 26.67,60.96 U28.3 | U30.3 26.67,54.61
  Bottom 0.152: U28.3 27.94,67.31 JP4.2
TO_REG2_2
  Top 0.152: 40.64,54.61 U45.3 R22.2 | 40.64,54.61 40.64,60.96 U44.3 | U46.3 40.64,54.61
  Bottom 0.152: U44.3 36.83,66.04 31.75,66.04 JP4.3
TO_REG2_3
  Top 0.152: U59.3 54.61,60.96 54.61,54.61 | 54.61,54.61 U60.3 R29.2 | U61.3 54.61,54.61
  Bottom 0.152: R29.2 54.61,57.15 54.61,63.5 48.26,69.85 41.91,69.85 41.91,68.58 JP4.4
VCC  (via drill 0.35)
  Top 0.152: 2.54,50.8 2.54,60.96 R9.1 3.81,64.77 R10.2 R11.1 R13.2 | 2.54,50.8 R7.2 | R8.2 2.54,40.64 | 2.54,40.64 2.54,50.8 | R6.2 2.54,30.48 | 2.54,30.48 2.54,40.64 | R5.2 2.54,12.7 2.54,30.48 | R1.2 16.51,12.7 16.51,30.48 | 16.51,30.48 R2.2 | 16.51,30.48 16.51,40.64 | 16.51,40.64 R4.2 | 16.51,40.64 16.51,50.8 | 16.51,50.8 R3.2 | 16.51,50.8 16.51,60.96 R12.1 17.78,64.77 R13.2 | R13.2 R14.1 31.75,64.77 | 31.75,64.77 R20.1 30.48,60.96 30.48,50.8 | 31.75,64.77 R21.2 R22.1 38.1,63.5 R30.2 | 30.48,50.8 R18.2 | R19.2 30.48,40.64 | 30.48,40.64 30.48,50.8 | 30.48,40.64 30.48,30.48 | 30.48,30.48 R17.2 | 30.48,30.48 30.48,12.7 R15.2 | R23.2 44.45,12.7 44.45,30.48 | 44.45,30.48 R24.2 | 44.45,30.48 44.45,40.64 | R26.2 44.45,40.64 | 44.45,40.64 44.45,50.8 | 44.45,50.8 R25.2 | 44.45,50.8 44.45,60.96 R27.1 R30.2 | R29.1 R28.2 46.99,64.77 R30.2 | v31.75,3.81 JP2.1
  Bottom 0.152: JP2.1 31.75,10.16 44.45,10.16 45.72,11.43 R23.2 | R16.2 v31.75,3.81
~CLK
  Top 0.152: U21.3 50.8,11.43 R16.1
  Bottom 0.152: R16.1 58.42,11.43 58.42,69.85 JP6.1
~LOAD  (via drill 0.35)
  Top 0.152: U62.3 45.72,68.58 R30.1 | v43.18,58.42 v43.18,62.23
  Bottom 0.152: U14.2 10.16,46.99 10.16,48.26 12.7,48.26 12.7,46.99 U22.2 24.13,46.99 24.13,48.26 26.67,48.26 26.67,46.99 U40.2 38.1,46.99 38.1,48.26 40.64,48.26 40.64,46.99 43.18,46.99 | 43.18,46.99 U55.2 | U62.3 43.18,67.31 44.45,67.31 44.45,64.77 43.18,64.77 v43.18,62.23 | v43.18,58.42 43.18,46.99
(copper drawn outside any net)
  shapes: Top area x2

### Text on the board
tNames: REGISTER2(OUT) | CARRY_OUT | ~CLK | 4-BIT BINARY COUNTER V1 | Q0 | Q1 | Q2 | Q3 | Q0 | Q0 | Q1 | Q2 | Q3 | B0 | B1 | B2 | B3 | VCC | GND | CARRY(IN) | LOAD | CLK_IN | RST | REGISTER1(IN) | BUS(IN) | CONTROL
